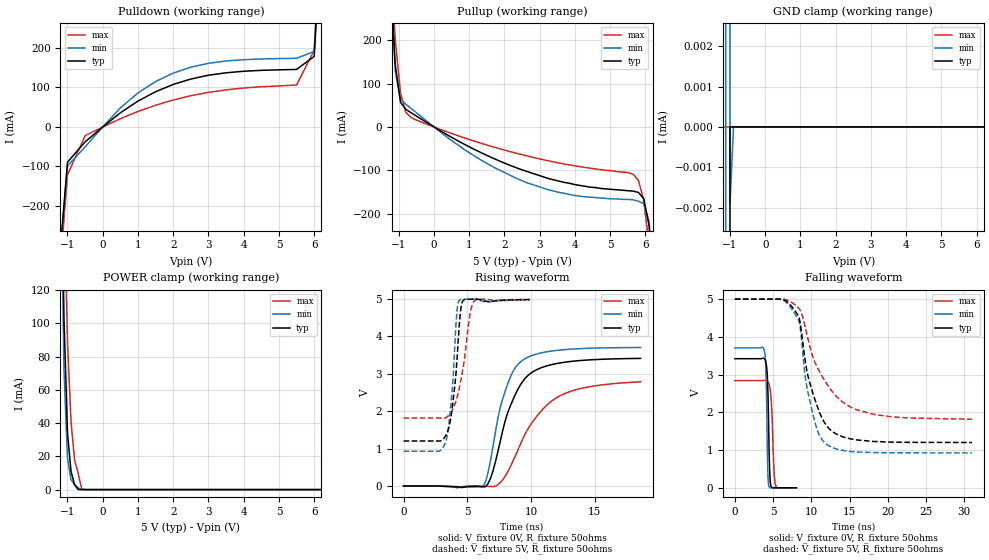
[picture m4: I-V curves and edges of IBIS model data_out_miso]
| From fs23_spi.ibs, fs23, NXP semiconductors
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|   Model data_out_miso
[Model]   data_out_miso
Model_type   Output
Polarity   Non-Inverting
Vmeas = 2.5
Cref = 2pF
Rref = 50
|   typ   min   max
C_comp   1.78p  1.17p  2.35p
||   typ   min   max
[Temperature Range]   27   -40   175
|   typ   min   max
[Voltage Range]   5V   4.8V   5.2V
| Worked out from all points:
|   slope of the pulldown table from 0 to 0.75 V, typ, clamps not added: 14.8 ohm
|   slope of the pullup table from 0 to 0.75 V, typ, clamps not added: 21.4 ohm
|   GND clamp passes 1 mA (typ) near -1.15 V on its own axis
|   POWER clamp passes 1 mA (typ) near -0.73 V on its own axis
|   rising waveform, V_fixture 0V, R_fixture 50ohms: 20-80 % time 1.98ns typ, 1.6ns min, 3.03ns max; typ from 0 V to 3.41 V
|   falling waveform, V_fixture 0V, R_fixture 50ohms: 20-80 % time 226ps typ, 189ps min, 318ps max; typ from 3.42 V to 0.005 V
|   rising waveform, V_fixture 5V, R_fixture 50ohms: 20-80 % time 589ps typ, 500ps min, 849ps max; typ from 1.2 V to 4.99 V
|   falling waveform, V_fixture 5V, R_fixture 50ohms: 20-80 % time 2.52ns typ, 1.89ns min, 4.06ns max; typ from 5 V to 1.2 V
[GND Clamp]
|Voltage   I(typ)   I(min)   I(max)
-5V       -6.37A     -6.63A     -5.6A
-1.4V     -18mA      -139mA     -700uA
-1.3V     -5mA       -80mA      55pA
-1.2V     -1.7mA     -10mA      55pA
-1.1V     -269uA     2.56mA     55pA
-1V       53pA       -1.9uA     55pA
-900mV    53pA       251pA      55pA
10V       53pA       251pA      55pA
[Power Clamp]
|Voltage   I(typ)   I(min)   I(max)
-5V       9.2A       9.8A       8.1A
-1.2V     236mA      211mA      305mA
-1.1V     103mA      72mA       178mA
-1V       34mA       19mA       89mA
-900mV    11mA       6mA        41mA
-800mV    3mA        3mA        18mA
-700mV    88uA       1mA        10mA
-600mV    14nA       14uA       664uA
-500mV    400pA      500pA      13uA
10V       400pA      500pA      36nA
[Pulldown]
|Voltage   I(typ)   I(min)   I(max)
-5V       -6.219A    -6.269A    -6.164A
-1.5V     -633.5mA   -631.5mA   -685mA
-1V       -89.37mA   -98.97mA   -121.2mA
-500mV    -37.87mA   -50.68mA   -22.23mA
500mV     35.84mA    48.22mA    20.9mA
1V        65.52mA    86.2mA     39.25mA
2V        107.8mA    136.5mA    68.29mA
3.5V      137.3mA    167.2mA    94.08mA
5.5V      145.8mA    174mA      106.4mA
6V        178.9mA    191.5mA    194.7mA
6.5V      959mA      1.031A     899.3mA
10V       9.419A     10.24A     8.261A
[Pullup]
-5V       9.379A     10.19A     8.226A
-1.25V    367mA      366mA      404mA
-1.1V     144mA      128mA      202mA
-950mV    56.7mA     63.8mA     78.1mA
-800mV    40.6mA     52.3mA     33.8mA
-650mV    32.7mA     42.6mA     21.6mA
1.15V     -52mA      -67.1mA    -32.8mA
2.65V     -103mA     -129mA     -67.1mA
5.65V     -148mA     -168mA     -109mA
5.95V     -165mA     -177mA     -168mA
6.1V      -226mA     -217mA     -270mA
10V       -6.255A    -6.31A     -6.188A
[Ramp]
R_load = 50ohms
|   typ   min   max
dV/dt_r   0.829/1e-9   0.445/1e-9   1.14/1e-9
dV/dt_f   7.127/1e-9   4.101/1e-9   8.299/1e-9
[Rising Waveform]
V_fixture = 0V
R_fixture = 50ohms
|Time   V(typ)   V(min)   V(max)
0s        17.2pV     428fV      422nV
6.2ns     -18.1mV    -24.7mV    -11.6mV
6.8ns     185mV      643mV      -13.4mV
7.4ns     919mV      1.812V     34.1mV
8ns       1.778V     2.565V     276mV
8.8ns     2.47V      3.181V     829mV
9.6ns     2.903V     3.418V     1.433V
11ns      3.188V     3.574V     2.081V
12.6ns    3.308V     3.646V     2.466V
18.6ns    3.413V     3.704V     2.787V
[falling Waveform]
V_fixture = 0V
R_fixture = 50ohms
|Time   V(typ)   V(min)   V(max)
0s        3.423V     3.708V     2.843V
3.8ns     3.433V     3.683V     2.846V
4.05ns    3.339V     3.228V     2.849V
4.25ns    2.965V     1.008V     2.83V
4.45ns    1.348V     56.3mV     2.762V
4.65ns    137mV      6.16mV     2.573V
4.85ns    12.7mV     3.52mV     2.005V
5.1ns     3.74mV     3.02mV     550mV
5.35ns    3.62mV     3.43mV     58.7mV
8.05ns    5.41mV     5.1mV      5.71mV
[Rising Waveform]
V_fixture = 5V
R_fixture = 50ohms
|Time   V(typ)   V(min)   V(max)
0s        1.204V     929mV      1.816V
3.3ns     1.343V     1.176V     1.825V
3.6ns     1.626V     1.777V     1.912V
3.9ns     2.317V     2.941V     2.083V
4.2ns     3.415V     4.726V     2.375V
4.4ns     4.439V     4.975V     2.666V
4.7ns     4.971V     4.995V     3.211V
5.2ns     4.996V     4.997V     4.574V
5.5ns     4.996V     4.997V     4.928V
9.9ns     4.987V     4.99V      4.979V
[falling Waveform]
V_fixture = 5V
R_fixture = 50ohms
|Time   V(typ)   V(min)   V(max)
0s        5V         5V         5V
6.1ns     4.998V     4.994V     5V
7.6ns     4.764V     4.691V     4.894V
8.5ns     4.428V     4.34V      4.722V
9.3ns     3.245V     2.817V     4.182V
10.4ns    2.39V      1.802V     3.365V
12.2ns    1.6V       1.129V     2.704V
14.6ns    1.327V     979mV      2.206V
18.1ns    1.232V     937mV      1.952V
31ns      1.204V     929mV      1.82V
